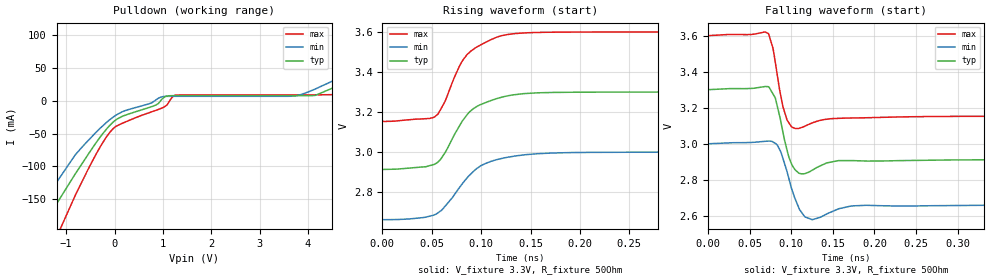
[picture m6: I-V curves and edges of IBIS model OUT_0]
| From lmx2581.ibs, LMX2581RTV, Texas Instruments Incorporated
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[Model]   OUT_0
Model_type   Open_drain
Polarity   Non-Inverting
Vmeas = 3.3
Vref = 3.3
Cref = 1pF
Rref = 50
|   typ   min   max
|   (nom PVT)   (slow PVT)   (fast PVT)
C_comp   0.269p   0.254p   0.289p
|C_comp (Hi state)   0.335p   0.327p   0.337p
|C_comp (Low state)   0.269p   0.254p   0.289p
[Voltage Range]   3.3   3   3.6
[Temperature Range]   27   125   -40
[Pullup Reference]   3.3   3   3.6
[Pulldown Reference]   0   0   0
[Power Clamp Reference]   3.3   3   3.6
[GND Clamp Reference]   0   0   0
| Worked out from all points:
|   slope of the pulldown table from 0 to 0.495 V, typ, clamps not added: 32.3 ohm
|   falling waveform, V_fixture 3.3V, R_fixture 50Ohm: 20-80 % time 11.1ps typ, 13ps min, 9.67ps max; typ from 3.3 V to 2.91 V
|   rising waveform, V_fixture 3.3V, R_fixture 50Ohm: 20-80 % time 31.4ps typ, 36.3ps min, 29ps max; typ from 2.91 V to 3.3 V
[Pulldown]
|   Voltage   I(typ)   I(min)   I(max)
-3.3V     -459mA     -398.5mA   -603.7mA
-2.191V   -304.3mA   -265.3mA   -399mA
-1.27V    -166.8mA   -134.1mA   -221.4mA
-1.181V   -154.8mA   -122.3mA   -204.8mA
-815.1mV  -111.6mA   -82.58mA   -144.5mA
-171.6mV  -43.57mA   -33.35mA   -55.51mA
155.1mV   -23.9mA    -16.93mA   -34.48mA
1.026V    5.278mA    6.515mA    -9.432mA
1.264V    7.736mA    6.756mA    8.56mA
3.67V     7.74mA     6.94mA     8.943mA
4.531V    19.9mA     30.72mA    9.326mA
6.6V      111.5mA    108.4mA    109.9mA
[Ramp]
R_load = 50
|   typ   min   max
dV/dt_r   0.232094/3.14171e-11   0.202663/3.6308e-11   0.268261/2.89968e-11
dV/dt_f   0.232101/1.10919e-11   0.202695/1.29594e-11   0.268279/9.67372e-12
[Falling Waveform]
V_fixture = 3.3V
V_fixture_min = 3V
V_fixture_max = 3.6V
R_fixture = 50Ohm
C_fixture = 0F
|   Time   V(typ)   V(min)   V(max)
0s        3.3V       3V         3.6V
72.64ps   3.316V     3.015V     3.61V
80.76ps   3.254V     3.002V     3.45V
89.81ps   3.066V     2.92V      3.207V
97.21ps   2.925V     2.804V     3.115V
104.8ps   2.855V     2.693V     3.085V
116.2ps   2.834V     2.595V     3.097V
125.2ps   2.854V     2.579V     3.116V
190.3ps   2.904V     2.659V     3.144V
900ps     2.913V     2.662V     3.153V
[Rising Waveform]
V_fixture = 3.3V
V_fixture_min = 3V
V_fixture_max = 3.6V
R_fixture = 50Ohm
C_fixture = 0F
|   Time   V(typ)   V(min)   V(max)
0s        2.913V     2.662V     3.153V
52.97ps   2.939V     2.687V     3.176V
56.47ps   2.951V     2.697V     3.191V
63.45ps   2.997V     2.729V     3.253V
77.94ps   3.13V      2.822V     3.429V
85.64ps   3.186V     2.87V      3.487V
104.1ps   3.246V     2.942V     3.547V
134.3ps   3.287V     2.98V      3.592V
210.3ps   3.299V     2.998V     3.6V
900ps     3.3V       3V         3.6V
